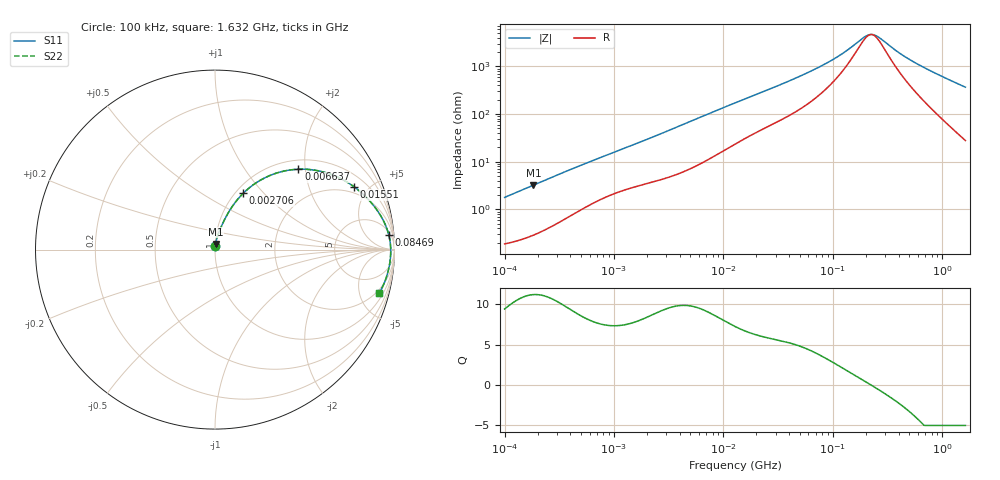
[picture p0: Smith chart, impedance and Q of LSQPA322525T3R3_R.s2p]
! LSQPA322525T3R3_R  S-PARAMETER MODEL  ( General Type )
! Model Generated by TAIYO YUDEN Corporation (http://www.ty-top.com)
! Version 2.0
! TAIYO YUDEN Control No. 100810NF25SB-FKC
! Copyright(c) 2007 TAIYO YUDEN CO.,LTD. All Rights Reserved.
! Product Description (link to TY-COMPAS)
! https://ds.yuden.co.jp/TYCOMPAS/or/detail?pn=LSQPA322525T3R3MR&u=M
! Products Name : Inductors
! Characteristics :
!  Inductance : 3.3 uH , SRF(min) : 160 MHz , DC Resistance(max) : 0.1235 Ohm
!  Rated Current : Saturation :2000 mA , Temp Rise : 1040 mA (40 degC)
!  Case Size : 3.2 x 2.5 / 0.126 x 0.098 [mm/inch] , Thickness : 2.5 / 0.098 [mm/inch]
!  (Conditions: Temperature = 25 degC , DC Bias Current/Voltage = 0A / 0V)
! External Node Assignments :
!  1  o---GGG---o  2
! GND o---------o GND
! Frequency Range : 0.1MHz  -  1631.998593MHz  [ 402 STEP ]
# MHz S RI R 50
! Freq[MHz].  S11 Real  S11 Imag  S21 Real  S21 Imag  S12 Real  S12 Imag  S22 Real  S22 Imag
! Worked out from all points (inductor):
!   401 points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, 100 kHz to 1.632 GHz, reference 50 ohm
!   read as one part in series: L = 2.82 uH near 105 kHz
!   highest Q = 11.2 at 183.4 kHz (marker M1), where L = 2.8 uH
!   self-resonance near 224.4 MHz
!   S11 on the Smith chart (normalised r, x): 100 kHz: 1.00, +0.04; 2.706 MHz: 1.08, +0.78; 6.637 MHz: 1.20, +1.84; 15.51 MHz: 1.60, +4.06; 84.69 MHz: 7, +22; 1.632 GHz: 1.56, -7.32
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0.1  0.0022 0.0177  0.9978 -0.0177  0.9978 -0.0177  0.0022 0.0177
0.183356  0.00391 0.0321  0.9961 -0.0321  0.9961 -0.0321  0.00391 0.0321
0.507727  0.0169 0.083  0.9831 -0.083  0.9831 -0.083  0.0169 0.083
1.339376  0.0627 0.1851  0.9373 -0.1851  0.9373 -0.1851  0.0627 0.1851
2.577871  0.1476 0.3038  0.8524 -0.3038  0.8524 -0.3038  0.1476 0.3038
2.705981  0.1576 0.314  0.8424 -0.314  0.8424 -0.314  0.1576 0.314
4.08663  0.2715 0.3969  0.7285 -0.3969  0.7285 -0.3969  0.2715 0.3969
6.637451  0.4648 0.4478  0.5352 -0.4478  0.5352 -0.4478  0.4648 0.4478
13.08855  0.7278 0.3808  0.2722 -0.3808  0.2722 -0.3808  0.7278 0.3808
15.51009  0.7761 0.3492  0.2239 -0.3492  0.2239 -0.3492  0.7761 0.3492
29.85196  0.8989 0.2256  0.1011 -0.2256  0.1011 -0.2256  0.8989 0.2256
64.86202  0.9598 0.1104  0.0402 -0.1104  0.0402 -0.1104  0.9598 0.1104
84.69158  0.9686 0.0807  0.0314 -0.0807  0.0314 -0.0807  0.9686 0.0807
121.8477  0.9753 0.0468  0.0247 -0.0468  0.0247 -0.0468  0.9753 0.0468
188.534  0.9787 0.0127  0.0213 -0.0127  0.0213 -0.0127  0.9787 0.0127
212.8377  0.979 0.00385  0.021 -0.00385  0.021 -0.00385  0.979 0.00385
228.8991  0.9791 -0.00145  0.0209 0.00145  0.0209 0.00145  0.9791 -0.00145
252.2152  0.9792 -0.00854  0.0208 0.00854  0.0208 0.00854  0.9792 -0.00854
329.3222  0.9786 -0.0287  0.0214 0.0287  0.0214 0.0287  0.9786 -0.0287
440.5575  0.9767 -0.0529  0.0233 0.0529  0.0233 0.0529  0.9767 -0.0529
618.654  0.972 -0.0868  0.028 0.0868  0.028 0.0868  0.972 -0.0868
1631.999  0.9149 -0.2435  0.0851 0.2435  0.0851 0.2435  0.9149 -0.2435
